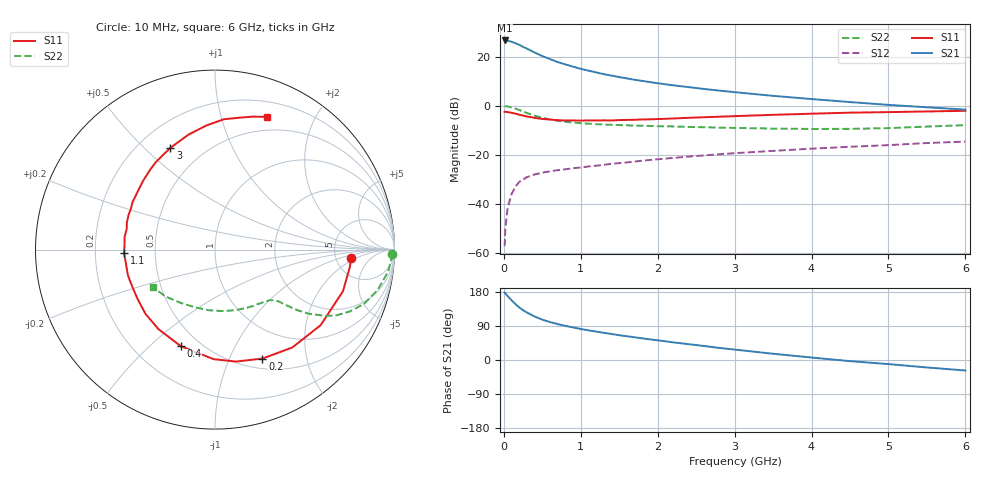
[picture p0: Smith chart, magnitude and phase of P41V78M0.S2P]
! SIEMENS Small Signal Semiconductors
! BFP182
! Si NPN RF Bipolar Junction Transistor in SOT143
! VCE = 1.75 V  IC = 8 mA
! Common Emitter S-Parameters:  March  1996
# GHz  S  MA  R  50
!  f  S11  S21  S12  S22
! GHz  MAG  ANG  MAG  ANG  MAG  ANG  MAG  ANG
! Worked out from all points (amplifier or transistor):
!   36 points, 10 MHz to 6 GHz, reference 50 ohm
!   highest |S21| = 26.6 dB at 10 MHz (marker M1)
!   |S21| within 3 dB of that: start of sweep to 277.1 MHz
!   unconditionally stable (mu >= 1): 1.222 GHz to 5.498 GHz
!   at 250 MHz: K = 0.29, MSG = 27.0 dB, |S12| = -30.0 dB
!   at 1.4 GHz: K = 1.07, MAG = 16.4 dB, |S12| = -23.6 dB
!   at 6 GHz: K = 0.93, MSG = 6.5 dB, |S12| = -14.5 dB
!   S11 on the Smith chart (normalised r, x): 10 MHz: 6.99, -1.54; 200 MHz: 0.62, -1.33; 400 MHz: 0.39, -0.63; 1.1 GHz: 0.33, -0.02; 3 GHz: 0.33, +0.60; 6 GHz: 0.35, +1.41
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0.01  0.76 -3.5  21.44 177.9  0.0014 82.7  0.985 -1.4
0.02  0.7574 -7.4  21.41 175.8  0.0033 81.3  0.9838 -3.0
0.05  0.7497 -18.0  21.22 168.5  0.0085 80.2  0.9724 -7.3
0.1  0.7237 -35.6  20.16 157.6  0.016 73.0  0.9323 -14.2
0.15  0.695 -51.7  18.84 147.6  0.0227 65.1  0.8826 -20.1
0.2  0.6622 -66.5  17.48 138.7  0.0284 60.4  0.8253 -24.7
0.25  0.6346 -79.4  15.91 131.4  0.0317 55.2  0.7684 -28.5
0.3  0.6106 -90.7  14.59 125.3  0.0356 51.4  0.7164 -31.0
0.4  0.5709 -109.5  12.19 114.7  0.0403 46.7  0.6352 -34.3
0.5  0.5437 -125.4  10.31 106.5  0.0438 43.3  0.5742 -36.2
0.6  0.5275 -137.2  8.967 100.2  0.0467 42.0  0.5301 -37.3
0.7  0.5114 -147.7  7.798 94.8  0.0492 40.7  0.4989 -38.1
0.9  0.5058 -163.5  6.284 86.0  0.054 40.4  0.4584 -39.1
1.1  0.5069 -177.7  5.217 78.2  0.0586 40.6  0.4344 -40.6
1.5  0.5141 162.7  3.858 65.4  0.0685 40.8  0.4077 -44.6
1.8  0.5301 150.1  3.22 57.1  0.0767 40.9  0.3948 -48.6
2.2  0.5546 136.2  2.627 46.6  0.0874 39.7  0.3817 -55.1
3  0.6189 113.7  1.904 27.5  0.1091 36.0  0.3568 -71.1
3.5  0.6581 102.8  1.6 16.5  0.1215 32.8  0.3451 -83.0
4.5  0.7283 86.0  1.196 -3.0  0.1473 26.1  0.3406 -109.7
5.5  0.7707 74.0  0.937 -19.7  0.1758 19.2  0.3795 -136.4
6  0.7942 68.6  0.84 -27.7  0.1875 14.5  0.4053 -149.0
